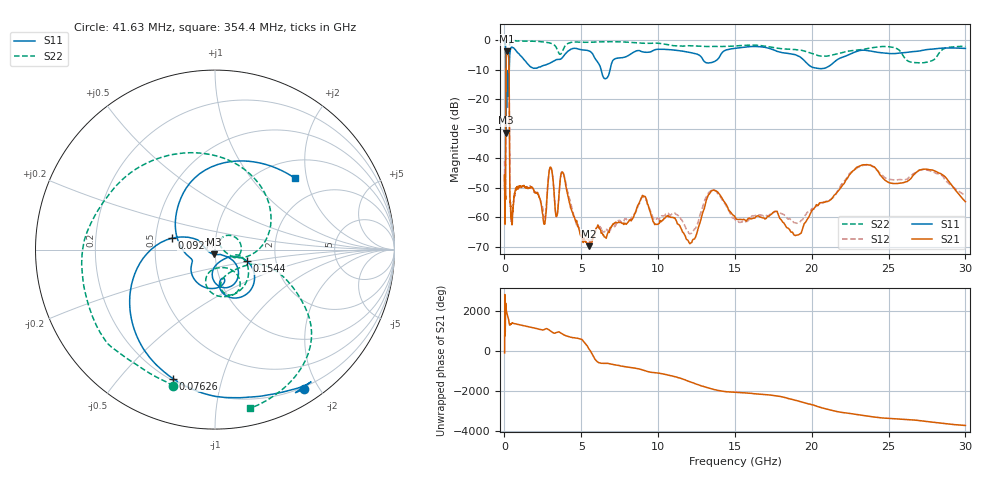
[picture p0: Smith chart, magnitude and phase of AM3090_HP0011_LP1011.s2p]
! Date/Time: Thu, Feb 28, 2019 1:56 PM
! Network Analyzer: Agilent Technologies E8364B Rev: A.07.50.67
! Sweep from 0.010 to 30.000 GHz, 1601 Points, Sweep Type: LOG
! Power Supply: 5.023 V, 0.002 A
# Hz S DB R 50
!freq MagS11 AngS11 MagS21 AngS21 MagS12 AngS12 MagS22 AngS22
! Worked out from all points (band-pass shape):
!   1601 points, 10 MHz to 30 GHz, reference 50 ohm
!   highest |S21| = -3.77 dB at 156 MHz (marker M1); lowest = -69.9 dB at 5.473 GHz (marker M2)
!   |S21| within 3 dB of the highest: 103.1 MHz to 284.4 MHz (181.3 MHz wide, 93.6 % of centre)
!   lowest |S11| = -31.4 dB at 100.9 MHz (marker M3), VSWR 1.06, Z = 49.4 - j2.62 ohm
!   |S11| at or under -10 dB: 91.55 MHz to 314.5 MHz (223 MHz wide, 110 % of centre); 6.288 GHz to 6.877 GHz (589 MHz wide, 8.95 % of centre)
!   |S22| runs from -28.8 to -0.1 dB; largest |S21 - S12| = 0.013
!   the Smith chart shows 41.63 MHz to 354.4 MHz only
!   S11 on the Smith chart (normalised r, x): 41.63 MHz: 0.17, -1.81; 76.26 MHz: 0.21, -0.71; 92.7 MHz: 0.61, +0.08; 154.4 MHz: 1.42, -0.19; 354.4 MHz: 1.39, +1.71
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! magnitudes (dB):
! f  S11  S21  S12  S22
! 10 MHz  -0.3  -45.9  -40.9  -0.7
! 38.04 MHz  -0.5  -61.6  -60.5  -1.7
! 41.63 MHz  -0.7  -59.7  -60.8  -2.0
! 76.26 MHz  -2.4  -46.0  -48.4  -4.5
! 92.7 MHz  -12.1  -15.0  -14.9  -12.1
! 100.9 MHz  -31.4  -7.5  -7.5  -28.2
! 116.7 MHz  -13.2  -5.0  -5.0  -17.9
! 144.7 MHz  -21.4  -3.8  -3.8  -19.1
! 154.4 MHz  -14.5  -3.8  -3.7  -16.2
! 156 MHz  -13.8  -3.8  -3.7  -15.7
! 288.7 MHz  -16.1  -7.4  -7.3  -15.4
! 354.4 MHz  -4.5  -52.8  -51.7  -0.9
! 550.5 MHz  -2.6  -57.0  -57.6  -0.3
! 2.084 GHz  -9.6  -51.9  -51.7  -0.5
! 2.597 GHz  -8.6  -62.4  -60.1  -0.7
! 2.972 GHz  -7.8  -43.1  -43.2  -1.0
! 3.402 GHz  -6.6  -59.5  -59.7  -2.9
! 3.798 GHz  -5.8  -44.9  -44.7  -3.5
! 5.473 GHz  -3.6  -69.9  -67.8  -0.8
! 7.926 GHz  -5.6  -62.5  -60.6  -0.7
! 23.36 GHz  -3.4  -42.3  -42.5  -3.2
! 30 GHz  -2.9  -54.8  -52.7  -2.2
